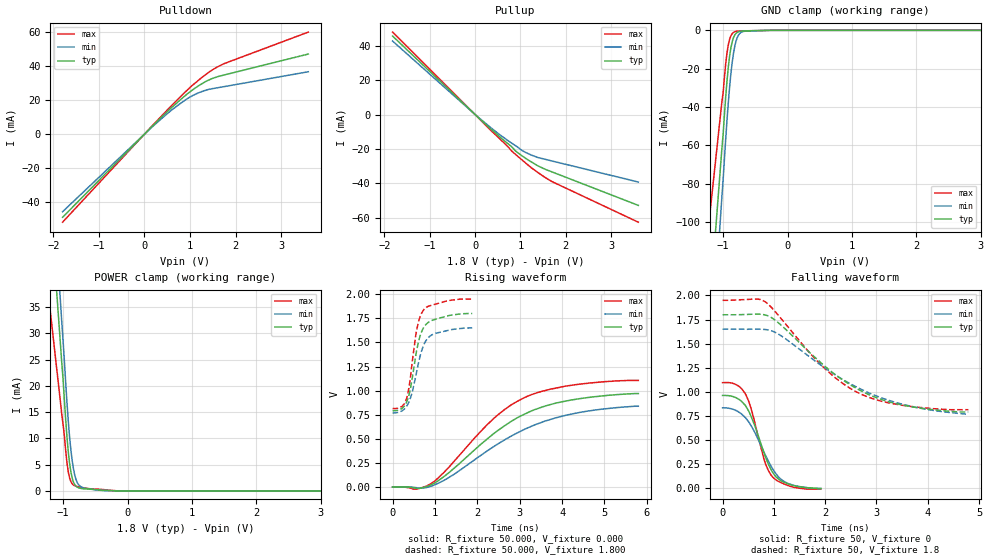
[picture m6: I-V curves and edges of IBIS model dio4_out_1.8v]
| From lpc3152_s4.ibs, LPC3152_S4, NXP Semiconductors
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[Model]   dio4_out_1.8v
Model_type Output
Vref=0.000E+00
Rref=1.000E+06
Cref=2.500E-11
Vmeas=9.000E-01
C_comp   1.080E-12   1.060E-12   1.100E-12
[Voltage Range]   1.800E+00   1.650E+00   1.950E+00
[POWER Clamp Reference]   1.800E+00   1.650E+00   1.950E+00
[GND Clamp Reference]   0.000E+00   0.000E+00   0.000E+00
[Pullup Reference]   1.800E+00   1.650E+00   1.950E+00
[Pulldown Reference]   0.000E+00   0.000E+00   0.000E+00
[Temperature Range]   25   85   -40
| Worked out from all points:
|   slope of the pulldown table from 0 to 0.27 V, typ, clamps not added: 37.4 ohm
|   slope of the pullup table from 0 to 0.27 V, typ, clamps not added: 41 ohm
|   GND clamp passes 1 mA (typ) near -0.78 V on its own axis
|   POWER clamp passes 1 mA (typ) near -0.81 V on its own axis
|   rising waveform, R_fixture 50.000, V_fixture 0.000: 20-80 % time 1.76ns typ, 1.94ns min, 1.57ns max; typ from 0 V to 0.969 V
|   falling waveform, R_fixture 50, V_fixture 0: 20-80 % time 411ps typ, 487ps min, 343ps max; typ from 0.962 V to -0.002 V
|   rising waveform, R_fixture 50.000, V_fixture 1.800: 20-80 % time 267ps typ, 297ps min, 228ps max; typ from 0.79 V to 1.8 V
|   falling waveform, R_fixture 50, V_fixture 1.8: 20-80 % time 1.44ns typ, 1.64ns min, 1.27ns max; typ from 1.8 V to 0.79 V
[GND Clamp]
-1.8V     -402.4mA   -477.2mA   -281.4mA
-1.02V    -61.84mA   -87.15mA   -37.46mA
-1V       -54.07mA   -77.69mA   -32.49mA
-960mV    -34.63mA   -56.56mA   -17.35mA
-940mV    -26.31mA   -46.78mA   -11.72mA
-920mV    -19.25mA   -37.77mA   -7.551mA
-880mV    -9.204mA   -22.72mA   -2.861mA
-840mV    -3.86mA    -12.1mA    -1.092mA
-800mV    -1.554mA   -5.647mA   -535.4uA
-760mV    -734.8uA   -2.404mA   -374uA
-660mV    -289.9uA   -451.2uA   -261.2uA
3.6V      0A         0A         0A
[Power Clamp]
-1.82V    161.3mA    177.2mA    99.25mA
-1.76V    151mA      170.3mA    95.5mA
-1.04V    27.58mA    35.69mA    16.71mA
-1V       21.05mA    28.35mA    12.57mA
-960mV    13.47mA    20.5mA     7.57mA
-920mV    7.417mA    13.24mA    3.594mA
-880mV    3.617mA    7.802mA    1.775mA
-840mV    1.686mA    4.229mA    1.109mA
-780mV    711.9uA    1.554mA    842.4uA
-720mV    462.3uA    763.8uA    674.2uA
-420mV    152.9uA    115.3uA    312.8uA
3.6V      0A         0A         0A
[Pullup]
-1.82V    45.6mA     42.71mA    47.91mA
80mV      -1.998mA   -1.832mA   -2.144mA
520mV     -12.44mA   -11.26mA   -13.51mA
820mV     -19.1mA    -16.88mA   -21.56mA
900mV     -21.37mA   -18.26mA   -23.37mA
1.04V     -24.11mA   -20.99mA   -26.52mA
1.38V     -29.78mA   -24.95mA   -33.59mA
1.72V     -33.61mA   -27.16mA   -39.31mA
3.6V      -52.83mA   -39.25mA   -62.59mA
[Pulldown]
-1.8V     -48.89mA   -45.62mA   -51.77mA
160mV     4.351mA    4.021mA    4.635mA
600mV     15.71mA    14.24mA    16.93mA
1.04V     25.7mA     22.42mA    28.41mA
1.4V      31.67mA    26.23mA    36.1mA
1.58V     33.54mA    27.14mA    39.18mA
1.76V     34.85mA    27.99mA    41.57mA
3.6V      47.09mA    36.68mA    60mA
[Rising Waveform]
R_fixture = 50.000
V_fixture = 0.000
V_fixture_min = 0.000
V_fixture_max = 0.000
|  time   V(typ)   V(min)   V(max)
0s        0V         0V         0V
565ps     -15.04mV   -7.704mV   -22.37mV
940ps     28.98mV    12.56mV    43.91mV
1.44ns    189.6mV    128.1mV    260.4mV
2.375ns   549.1mV    415.3mV    705.4mV
2.805ns   681.6mV    528.9mV    853.1mV
3.18ns    769.5mV    611.2mV    941.1mV
3.72ns    854.4mV    699.6mV    1.014V
4.415ns   916.2mV    773.2mV    1.067V
5.8ns     969.3mV    837.5mV    1.106V
[Falling Waveform]
R_fixture = 50
V_fixture = 0
V_fixture_min = 0
V_fixture_max = 0
0s        962.1mV    834.3mV    1.095V
240ps     944mV      811.1mV    1.08V
440ps     861.1mV    734.7mV    983.6mV
570ps     726.8mV    635.5mV    799.9mV
815ps     353.6mV    364.6mV    287.1mV
900ps     240.1mV    272.5mV    175.8mV
980ps     160.5mV    197.2mV    113.3mV
1.115ns   85.56mV    104mV      63.2mV
1.28ns    43.6mV     47.8mV     26.11mV
1.915ns   -2.413mV   -4.96mV    -10.66mV
[Rising Waveform]
R_fixture = 50.000
V_fixture = 1.800
V_fixture_min = 1.650
V_fixture_max = 1.950
|  time   V(typ)   V(min)   V(max)
0s        790.3mV    768.2mV    814.2mV
215ps     813.1mV    787.9mV    833.8mV
330ps     880.3mV    836mV      915.7mV
425ps     1.029V     926.4mV    1.15V
570ps     1.42V      1.199V     1.631V
645ps     1.56V      1.349V     1.761V
725ps     1.648V     1.463V     1.833V
835ps     1.705V     1.546V     1.873V
990ps     1.737V     1.591V     1.895V
1.88ns    1.8V       1.65V      1.95V
[Falling Waveform]
R_fixture = 50
V_fixture = 1.8
V_fixture_min = 1.65
V_fixture_max = 1.95
0s        1.8V       1.65V      1.95V
675ps     1.807V     1.65V      1.963V
825ps     1.799V     1.647V     1.936V
1.165ns   1.681V     1.573V     1.745V
1.99ns    1.266V     1.249V     1.243V
2.33ns    1.127V     1.131V     1.091V
2.705ns   1.008V     1.025V     973.8mV
3.08ns    923.4mV    940.8mV    904.3mV
3.515ns   861.5mV    869.6mV    858.9mV
4.79ns    790.3mV    768.2mV    814.2mV
[Ramp]
dV/dt_r   5.7872E-01/1.7570E-09   5.0357E-01/1.9462E-09   6.6336E-01/1.5645E-09
dV/dt_f   6.0579E-01/1.4344E-09   5.2910E-01/1.6388E-09   6.8149E-01/1.2702E-09
R_load = 50
